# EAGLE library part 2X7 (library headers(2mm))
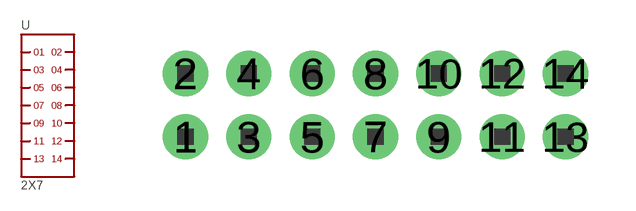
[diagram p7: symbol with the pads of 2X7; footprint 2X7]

Designator prefix -

## 2X7  [2X7]
1  1
2  2
3  3
4  4
5  5
6  6
7  7
8  8
9  9
10  10
11  11
12  12
13  13
14  14

## Footprint 2X7 (pad centres in mm)
drill 0.8 pad 1.422: 1 -6,-1; 2 -6,1; 3 -4,-1; 4 -4,1; 5 -2,-1; 6 -2,1; 7 0,-1; 8 0,1; 9 2,-1; 10 2,1; 11 4,-1; 12 4,1; 13 6,-1; 14 6,1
